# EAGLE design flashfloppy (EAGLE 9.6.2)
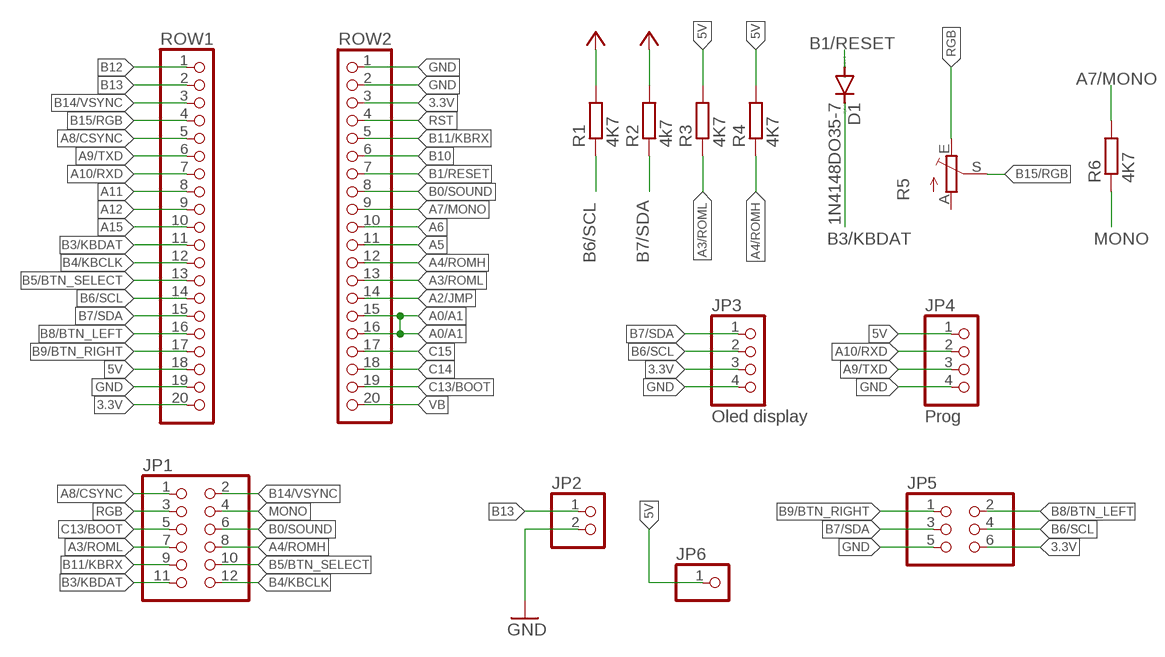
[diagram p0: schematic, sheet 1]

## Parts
D1  1N4148DO35-7  [DO35-7]
JP1  PINHD-2X6/90  [2X06/90]
JP2  PINHD-1X2  [1X02]
JP3  Oled display  PINHD-1X4/90  [1X04/90]
JP4  Prog  PINHD-1X4  [1X04]
JP5  PINHD-2X3  [2X03]
JP6  PINHD-1X1  [1X01]
R1  4K7  R-EU_0204/5  [0204/5]
R2  4k7  R-EU_0204/5  [0204/5]
R3  4K7  R-EU_0204/5  [0204/5]
R4  4K7  R-EU_0204/5  [0204/5]
R5  TRIM_EU-CA6V  [CA6V]
R6  4K7  R-EU_0204/5  [0204/5]
ROW1  PINHD-1X20  [1X20]
ROW2  PINHD-1X20  [1X20]

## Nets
3.3V: JP3.3 JP5.6 R1.2 R2.2 ROW1.20 ROW2.3 ; supply symbol labelled VCC
5V: JP4.1 JP6.1 R3.2 R4.2 ROW1.18
A0/A1: ROW2.15 ROW2.16
A2/JMP: ROW2.14
A3/ROML: JP1.7 R3.1 ROW2.13
A4/ROMH: JP1.8 R4.1 ROW2.12
A5: ROW2.11
A6: ROW2.10
A7/MONO: R6.2 ROW2.9
A8/CSYNC: JP1.1 ROW1.5
A9/TXD: JP4.3 ROW1.6
A10/RXD: JP4.2 ROW1.7
A11: ROW1.8
A12: ROW1.9
A15: ROW1.10
B0/SOUND: JP1.6 ROW2.8
B1/RESET: D1.A ROW2.7
B3/KBDAT: D1.C JP1.11 ROW1.11
B4/KBCLK: JP1.12 ROW1.12
B5/BTN_SELECT: JP1.10 ROW1.13
B6/SCL: JP3.2 JP5.4 R1.1 ROW1.14
B7/SDA: JP3.1 JP5.3 R2.1 ROW1.15
B8/BTN_LEFT: JP5.2 ROW1.16
B9/BTN_RIGHT: JP5.1 ROW1.17
B10: ROW2.6
B11/KBRX: JP1.9 ROW2.5
B12: ROW1.1
B13: JP2.1 ROW1.2
B14/VSYNC: JP1.2 ROW1.3
B15/RGB: R5.S ROW1.4
C13/BOOT: JP1.5 ROW2.19
C14: ROW2.18
C15: ROW2.17
GND: JP2.2 JP3.4 JP4.4 JP5.5 ROW1.19 ROW2.1
MONO: JP1.4 R6.1
N$1: ROW2.2
RGB: JP1.3 R5.E
RST: ROW2.4
VB: ROW2.20
Unconnected: R5.A

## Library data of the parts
D1 = diode:1N4148: DIODE
JP1 = pinhead:PINHD-2X6: PIN HEADER
JP2 = pinhead:PINHD-1X2: PIN HEADER
JP3 JP4 = pinhead:PINHD-1X4: PIN HEADER
JP5 = pinhead:PINHD-2X3: PIN HEADER
JP6 = pinhead:PINHD-1X1: PIN HEADER
R1-R4 R6 = rcl:R-EU_: RESISTOR, European symbol; SPICEPREFIX: R
R5 = pot:TRIM_EU-: POTENTIOMETER
ROW1 ROW2 = pinhead:PINHD-1X20: PIN HEADER

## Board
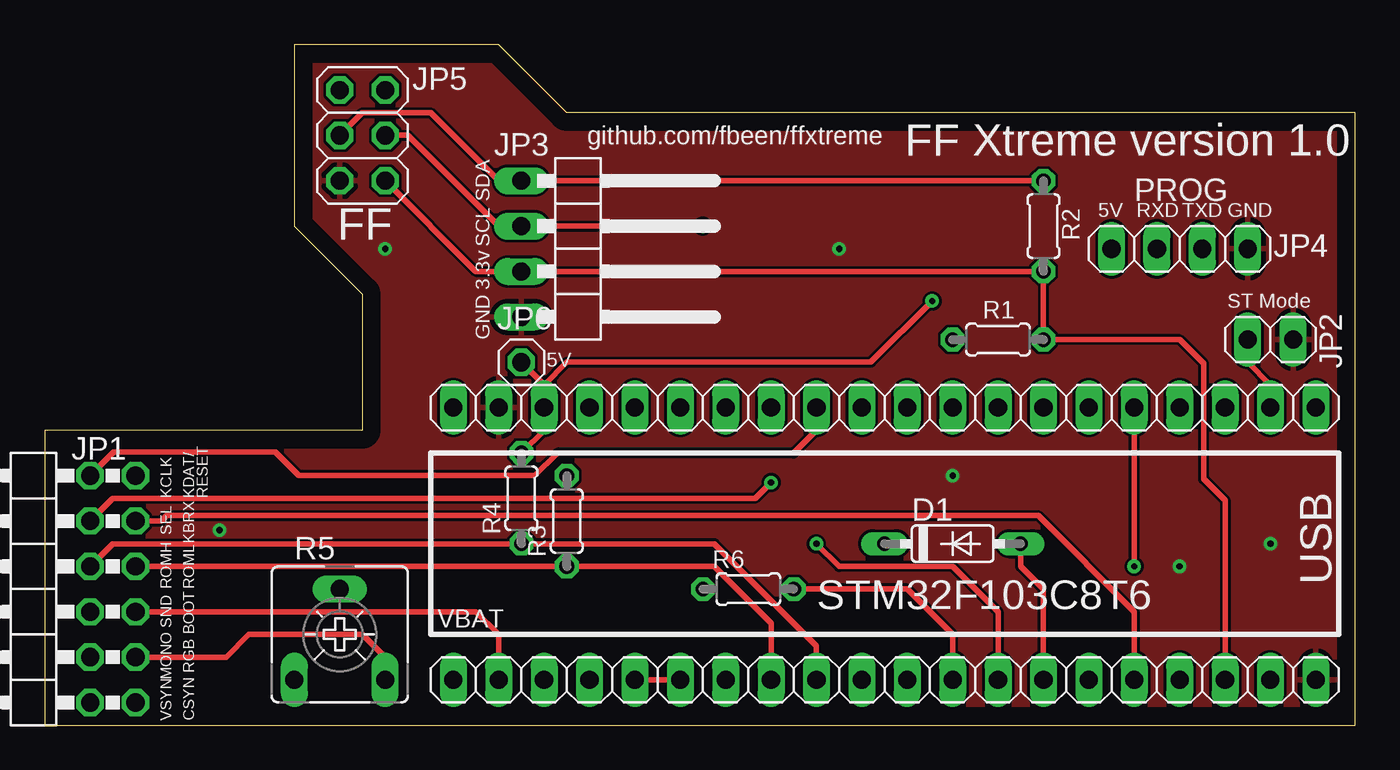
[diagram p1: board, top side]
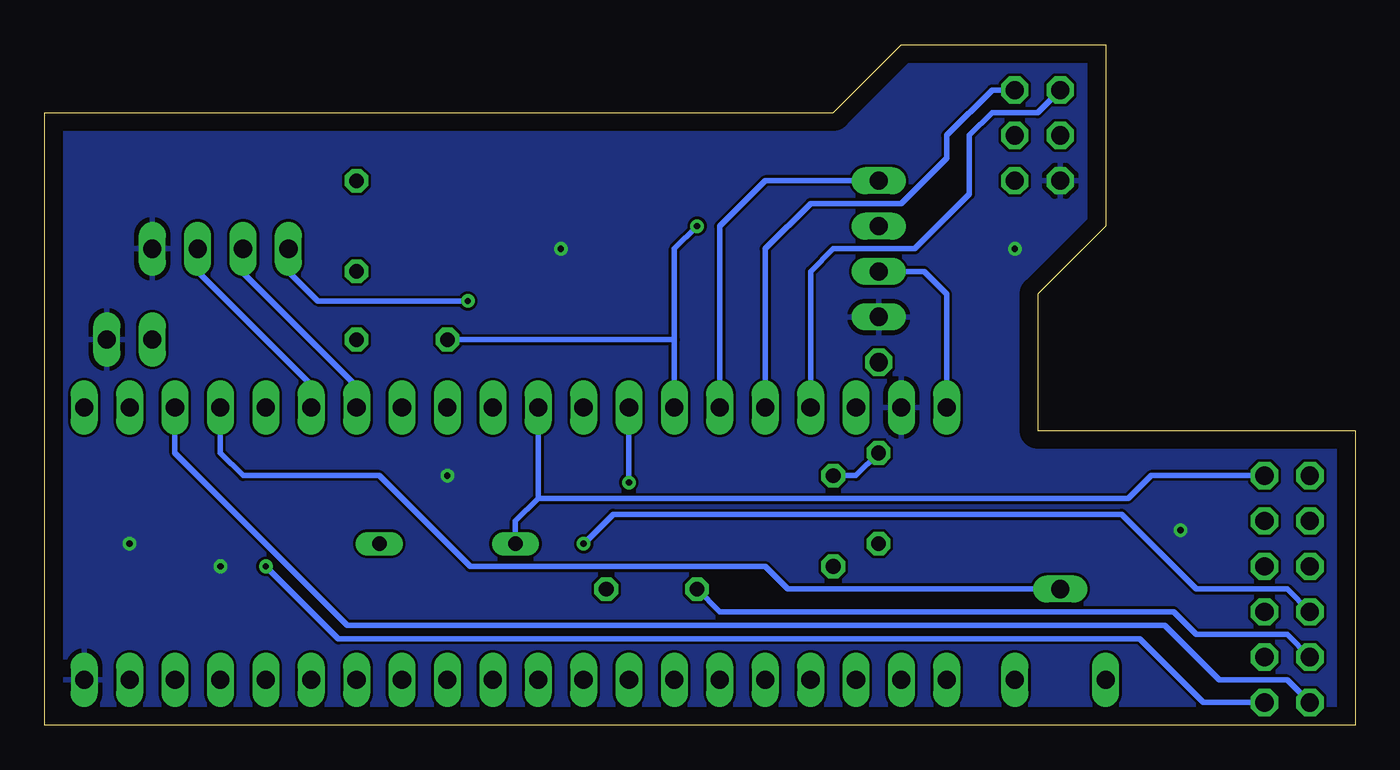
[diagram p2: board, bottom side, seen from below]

Size 73.33 x 38.1 mm. Coordinates in mm from the lower left corner, seen from the top.
Outline: 0,0 73.33,0 73.33,34.28 29.21,34.29 25.4,38.1 13.97,38.1 13.97,27.94 17.78,24.13 17.77,16.5 0,16.5 0,0
Copper layers (1*16): Top 0.035mm / dielectric 1.5mm / Bottom 0.035mm
Design rules "default": minimum track width 6mil, minimum drill 0.35mm, track to track 6mil, track to pad 6mil, pad to pad 6mil, via to via 6mil, smd to smd 6mil, copper to edge 40mil, drill to drill 6mil, minimum pad ring 10mil, minimum via ring 8mil, stop-mask expansion 4mil, vias tented up to drill 0mil, thermal gap 10mil

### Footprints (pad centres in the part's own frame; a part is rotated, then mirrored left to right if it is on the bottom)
DO35-7 = drill 0.813 long: A 3.81,0; C -3.81,0
2X06/90 = drill 1.016 octagon: 1 -6.35,-6.35; 2 -6.35,-3.81; 3 -3.81,-6.35; 4 -3.81,-3.81; 5 -1.27,-6.35; 6 -1.27,-3.81; 7 1.27,-6.35; 8 1.27,-3.81; 9 3.81,-6.35; 10 3.81,-3.81; 11 6.35,-6.35; 12 6.35,-3.81
1X02 = drill 1.016 long: 1 -1.27,0; 2 1.27,0
1X04/90 = drill 1.016 long: 1 -3.81,-3.81; 2 -1.27,-3.81; 3 1.27,-3.81; 4 3.81,-3.81
1X04 = drill 1.016 long: 1 -3.81,0; 2 -1.27,0; 3 1.27,0; 4 3.81,0
2X03 = drill 1.016 octagon: 1 -2.54,-1.27; 2 -2.54,1.27; 3 0,-1.27; 4 0,1.27; 5 2.54,-1.27; 6 2.54,1.27
1X01 = drill 1.016 octagon: 1 0,0
0204/5 = drill 0.813 octagon: 1 -2.54,0; 2 2.54,0
CA6V = drill 1.016 long: A -2.54,-2.54; E 2.54,-2.54; S 0,2.54
1X20 = drill 1.016 long: 1 -24.13,0; 2 -21.59,0; 3 -19.05,0; 4 -16.51,0; 5 -13.97,0; 6 -11.43,0; 7 -8.89,0; 8 -6.35,0; 9 -3.81,0; 10 -1.27,0; 11 1.27,0; 12 3.81,0; 13 6.35,0; 14 8.89,0; 15 11.43,0; 16 13.97,0; 17 16.51,0; 18 19.05,0; 19 21.59,0; 20 24.13,0

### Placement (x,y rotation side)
D1  50.8,10.16 0 top
JP1  -1.27,7.62 90 top
JP2  68.58,21.59 0 top
JP3  30.48,26.67 270 top
JP4  63.5,26.67 0 top
JP5  17.78,33.02 270 top
JP6  26.67,20.32 0 top
R1  53.34,21.59 0 top
R2  55.88,27.94 270 top
R3  29.21,11.43 90 top
R4  26.67,12.7 90 top
R5  16.51,5.08 0 top
R6  39.37,7.62 0 top
ROW1  46.99,17.78 180 top
ROW2  46.99,2.54 180 top

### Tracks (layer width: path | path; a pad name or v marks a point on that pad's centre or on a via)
3.3V
  Top 0.305: ROW2.3 66.04,12.59 64.85,13.78 64.85,20.24 63.5,21.59 R1.2 R2.2 JP3.3 24.13,25.4 JP5.6
  Bottom 0.305: ROW1.20 22.86,24.13 24.13,25.4 JP3.3
5V  (via drill 0.35)
  Top 0.305: R4.2 27.94,16.51 ROW1.18 27.94,19.05 | 27.94,19.05 29.21,20.32 46.23,20.32 v49.66,23.75 | JP6.1 27.94,19.05
  Bottom 0.305: R4.2 27.94,13.97 R3.2 | JP4.1 59.69,25.4 58.04,23.75 v49.66,23.75
A0/A1
  Top 0.305: ROW2.16 ROW2.15
A3/ROML
  Top 0.305: JP1.7 R3.1 37.47,8.89 40.64,5.71 ROW2.13
A4/ROMH
  Top 0.305: JP1.8 3.81,10.16 R4.1 37.47,10.16 43.18,4.45 ROW2.12
A7/MONO
  Top 0.305: ROW2.9 50.8,5.08 48.26,7.62 R6.2
A8/CSYNC  (via drill 0.35)
  Top 0.305: v60.96,8.89 ROW1.5
  Bottom 0.305: JP1.1 8.51,1.27 12.07,4.83 56.9,4.83 v60.96,8.89
A9/TXD
  Bottom 0.305: JP4.3 64.77,25.4 58.42,19.05 ROW1.6
A10/RXD
  Bottom 0.305: JP4.2 62.23,25.3 55.88,18.96 ROW1.7
B0/SOUND  (via drill 0.35)
  Top 0.305: v43.18,10.16 44.45,8.89 50.8,8.89 53.34,6.35 ROW2.8
  Bottom 0.305: JP1.6 3.81,7.62 8.89,7.62 13.08,11.81 41.53,11.81 v43.18,10.16
B1/RESET
  Top 0.305: ROW2.7 55.88,7.62 54.61,8.89 D1.A
B3/KBDAT
  Bottom 0.305: JP1.11 11.43,13.97 12.7,12.7 45.72,12.7 | D1.C 46.99,11.43 45.72,12.7 | ROW1.11 45.72,12.7
B4/KBCLK
  Top 0.305: ROW1.12 43.18,16.51 41.91,15.24 28.7,15.24 27.43,13.97 14.21,13.97 12.89,15.29 3.86,15.29 JP1.12
B5/BTN_SELECT  (via drill 0.35)
  Top 0.305: JP1.10 3.81,12.7 39.75,12.7 v40.64,13.59
  Bottom 0.305: ROW1.13 v40.64,13.59
B6/SCL  (via drill 0.35)
  Top 0.305: v36.83,27.94 JP3.2 25.4,27.94 20.32,33.02 JP5.4
  Bottom 0.305: R1.1 38.1,21.59 ROW1.14 38.1,26.67 v36.83,27.94
B7/SDA
  Top 0.305: R2.1 JP3.1 25.4,30.48 21.59,34.29 17.78,34.29 JP5.3
  Bottom 0.305: JP3.1 33.02,30.48 35.56,27.94 ROW1.15
B8/BTN_LEFT
  Bottom 0.305: ROW1.16 33.02,26.67 30.48,29.21 25.4,29.21 22.86,31.75 22.86,33.02 20.32,35.56 JP5.2
B9/BTN_RIGHT
  Bottom 0.305: ROW1.17 30.48,25.4 29.21,26.67 24.64,26.67 21.59,29.72 21.59,33.02 20.32,34.29 17.78,34.29 JP5.1
B11/KBRX
  Top 0.305: ROW2.5 60.96,6.35 55.58,11.73 6.83,11.73 6.53,11.43 JP1.9
B13
  Top 0.305: ROW1.2 68.58,19.05 67.31,20.32 JP2.1
B14/VSYNC
  Bottom 0.305: JP1.2 3.81,2.54 7.62,2.54 10.67,5.59 56.39,5.59 66.04,15.24 ROW1.3
B15/RGB
  Bottom 0.305: ROW1.4 63.5,15.24 62.23,13.97 54.61,13.97 49.53,8.89 33.02,8.89 31.75,7.62 R5.S
C13/BOOT
  Top 0.305: JP1.5 24.13,6.35 25.4,5.08 ROW2.19
GND  (via drill 0.35)
  other vias: 63.5,8.89 68.58,10.16 50.8,13.97 44.45,26.67 9.78,10.92 19.05,26.67
  pour Bottom: 0,16.51 17.78,16.51 17.78,24.13 13.97,27.94 13.97,38.1 25.4,38.1 29.21,34.29 73.66,34.29 73.66,0 0,0
  pour Top: 0,16.51 17.78,16.51 17.78,24.13 13.97,27.94 13.97,38.1 25.4,38.1 29.21,34.29 73.66,34.29 73.66,0 0,0
MONO
  Bottom 0.305: JP1.4 3.81,5.08 8.89,5.08 10.16,6.35 35.56,6.35 R6.1
RGB
  Top 0.305: R5.E 19.05,3.81 17.78,5.08 11.43,5.08 10.16,3.81 JP1.3

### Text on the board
tNames: github.com/fbeen/ffxtreme | FF Xtreme version 1.0 | SDA | PROG | 5V | RXD | TXD | GND | FF | SCL | 3.3v | ST Mode | GND | 5V | KCLK | KDAT/ | RESET | SEL | KBRX | ROMH | ROML | USB | STM32F103C8T6 | SND | VBAT | BOOT | MONO | RGB | VSYN | CSYN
